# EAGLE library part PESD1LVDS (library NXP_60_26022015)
ESD protection for in-vehicle ultra high-speed interfaces The device is designed to protect in-vehicle ultra high-speed interfaces in automotive applications, such as Low-Voltage Differential Signaling (LVDS), High-Definition Multimedia Interface (HDMI) and DisplayPort interfaces against ElectroStatic Discharge (ESD). AAL Eindhoven MK
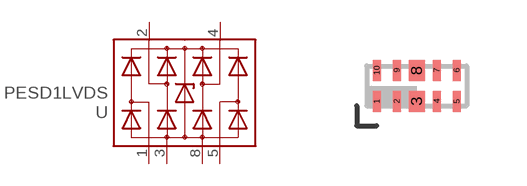
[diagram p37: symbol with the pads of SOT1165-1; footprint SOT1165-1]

Designator prefix -

## PESD1LVDS  [SOT1165-1]
1  CH1-  pas
2  CH1+  pas
3  GND  pwr
4  CH2-  pas
5  CH2+  pas
8  GND  pwr

## Footprint SOT1165-1 (pad centres in mm)
SOT1165-1 XSON10: plastic, extremely thin small outline package; no leads; 10 terminals; body 1 x 2.5 x 0.5 mm JEDEC: -- IEC: --
smd 0.2 x 0.525: 1 -1,-0.388; 2 -0.5,-0.388; 4 0.5,-0.388; 5 1,-0.388; 6 1,0.388; 7 0.5,0.388; 9 -0.5,0.388; 10 -1,0.388
smd 0.4 x 0.525: 3 0,-0.388; 8 0,0.388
